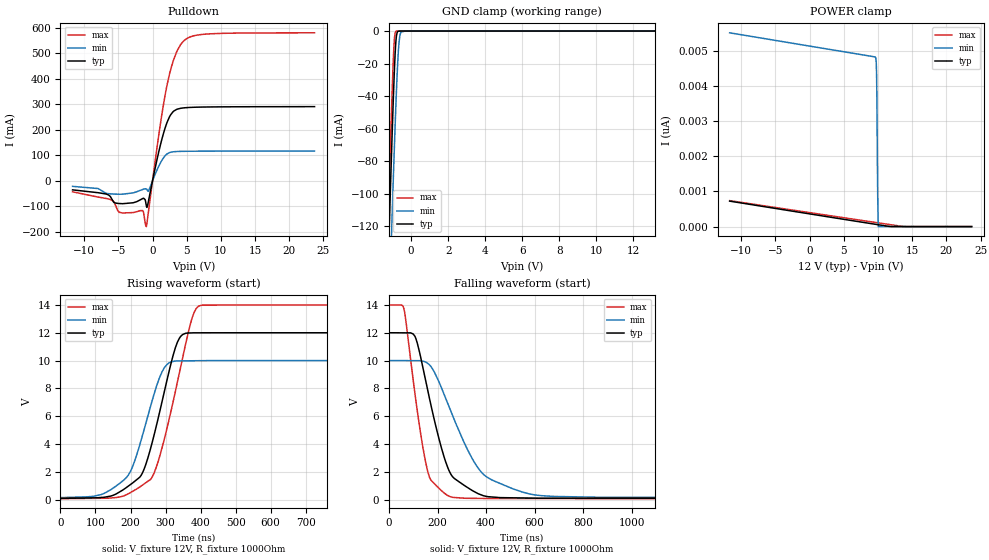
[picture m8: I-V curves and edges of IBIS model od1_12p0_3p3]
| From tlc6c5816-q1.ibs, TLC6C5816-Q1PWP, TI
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|   od1_12p0_3p3 Model
[Model]   od1_12p0_3p3
Model_type   Open_drain
Polarity   Inverting
Vmeas = 6
Vref = 12
Cref = 2pF
Rref = 1000
|   typ   min   max
C_comp   3.695pF   3.324pF   3.747pF
| Where Nom  PVT is Nominal Process, 12.0V, 27C
|   Fast PVT is Strong Process,  14.0V, -40C
|   Slow PVT is Weak Process,   10.0V, 150C
[Voltage Range]   12   10   14
|Junction Temperature
[Temperature Range]   27   150   -40
[Pullup Reference]   12   10   14
[Pulldown Reference]   0   -0   0
[Power Clamp Reference]   12   10   14
[GND Clamp Reference]   0   0   0
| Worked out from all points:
|   slope of the pulldown table from 0 to 1.8 V, typ, clamps not added: 8.87 ohm
|   GND clamp passes 1 mA (typ) near -0.76 V on its own axis
|   falling waveform, V_fixture 12V, R_fixture 1000Ohm: 20-80 % time 101ns typ, 158ns min, 67.9ns max; typ from 12 V to 0.09 V
|   rising waveform, V_fixture 12V, R_fixture 1000Ohm: 20-80 % time 71.1ns typ, 71.3ns min, 77.4ns max; typ from 0.09 V to 12 V
[Pulldown]
|   Voltage   I(typ)   I(min)   I(max)
-11.7V    -35.57mA   -21.83mA   -43.12mA
-6.107V   -64.35mA   -51.19mA   -73.95mA
-4.868V   -88.99mA   -52.59mA   -123.4mA
-1.434V   -69.39mA   -33.88mA   -116.7mA
-903mV    -98.24mA   -31.97mA   -179.3mA
-584.4mV  -77.91mA   -40.06mA   -119.1mA
902.4mV   112.3mA    56.61mA    176.9mA
2V        219.3mA    102.4mA    358.1mA
3.133V    273.4mA    113.8mA    477.6mA
4.513V    285.3mA    115.4mA    546.4mA
8.089V    289mA      116mA      574.8mA
23.7V     290.3mA    116.4mA    579.3mA
[GND Clamp]
|   Voltage   I(typ)   I(min)   I(max)
-11.7V    -5.142A    -4.912A    -5.294A
-1.257V   -147.7mA   -196.2mA   -122.2mA
-1.115V   -94.13mA   -143.7mA   -67.68mA
-1.045V   -68.45mA   -118.2mA   -42.16mA
-973.8mV  -44.18mA   -93.26mA   -19.47mA
-903mV    -22.64mA   -69.32mA   -4.129mA
-832.2mV  -7.051mA   -46.92mA   -263.1uA
-796.8mV  -2.903mA   -36.59mA   -56.31uA
-690.6mV  -89.96uA   -11.86mA   -687nA
-619.8mV  -7.619uA   -3.44mA    -55.01nA
-336.6mV  -444.4pA   -3.796uA   -12.88pA
23.7V     0A         0A         0A
[POWER Clamp]
|   Voltage   I(typ)   I(min)   I(max)
-11.7V    723.7pA    5.506nA    737.5pA
9.611V    65.75pA    4.814nA    118.3pA
9.717V    62.54pA    4.73nA     115.2pA
9.752V    61.47pA    4.619nA    114.2pA
9.788V    60.4pA     4.382nA    113.2pA
9.823V    59.33pA    3.921nA    112.2pA
9.859V    58.26pA    3.178nA    111.1pA
9.929V    56.12pA    1.456nA    109.1pA
9.965V    55.05pA    778.7pA    108.1pA
10.04V    52.91pA    0A         106pA
13.96V    0A         0A         455fA
23.7V     0A         0A         0A
[Ramp]
R_load = 1000
|   typ   min   max
dV/dt_r   7.14581/7.10699e-08   5.91306/7.13446e-08   8.35899/7.73987e-08
dV/dt_f   7.14583/1.00313e-07   5.91309/1.57528e-07   8.35901/6.788e-08
[Falling Waveform]
V_fixture = 12V
V_fixture_min = 10V
V_fixture_max = 14V
R_fixture = 1000Ohm
C_fixture = 0F
|   Time   V(typ)   V(min)   V(max)
0s        12V        10V        14V
61.37ns   11.99V     9.996V     13.73V
107.9ns   11.7V      9.992V     7.493V
139.7ns   9.493V     9.952V     3.75V
167ns     7.258V     9.689V     1.592V
216.3ns   3.703V     8.028V     642.5mV
256.8ns   1.774V     6.277V     187.3mV
388.4ns   286mV      1.832V     86.72mV
598.4ns   110.5mV    348.4mV    75.42mV
2.5us     90.28mV    144.8mV    68.31mV
[Rising Waveform]
V_fixture = 12V
V_fixture_min = 10V
V_fixture_max = 14V
R_fixture = 1000Ohm
C_fixture = 0F
|   Time   V(typ)   V(min)   V(max)
0s        90.28mV    144.8mV    68.31mV
115.9ns   156.5mV    361.5mV    99mV
187.1ns   849.7mV    1.554V     340.2mV
230.2ns   1.741V     4.265V     976.3mV
260.3ns   3.963V     6.985V     1.563V
296.5ns   7.761V     9.486V     4.358V
333.8ns   11.32V     9.976V     8.45V
373.7ns   11.99V     9.985V     12.88V
401.8ns   12V        9.991V     13.97V
2.5us     12V        10V        14V
